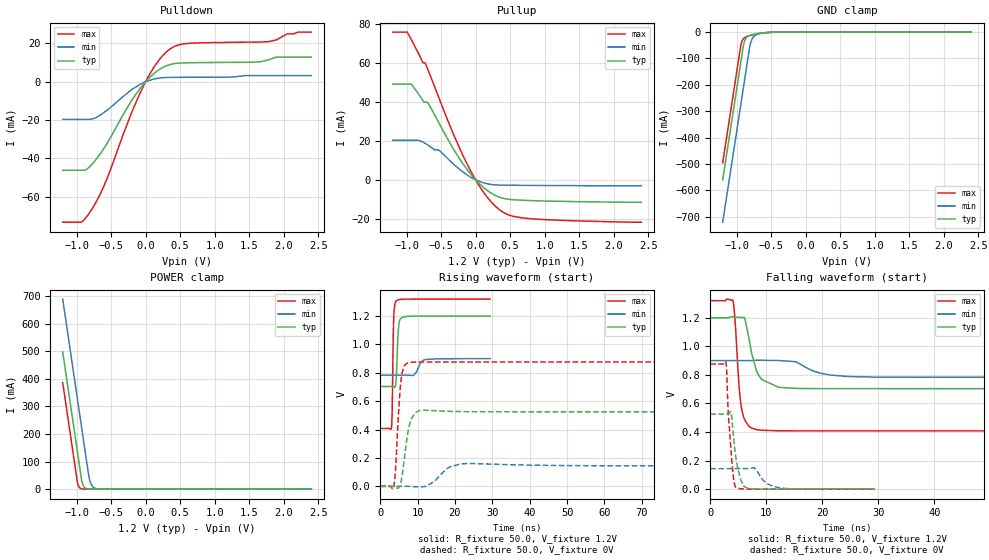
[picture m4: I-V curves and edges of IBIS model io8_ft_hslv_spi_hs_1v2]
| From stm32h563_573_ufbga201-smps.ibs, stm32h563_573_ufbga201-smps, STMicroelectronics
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[Model]   io8_ft_hslv_spi_hs_1v2
Model_type I/O
Polarity   Non-Inverting
Enable   Active-Low
| CAP_THRESHOLD on pad IOFT is "UDTCAPC" :
| Rising=20.0% of vddiom   Falling=80.0% of vddiom
| C_comp min and max val. don't necessarily correlate with the min and max pvt
| but are the smallest and greatest pad capacitance found.
| var   typ   min   max
C_comp   4.03050pF  3.93195pF  4.03600pF
|C_comp_pullup   2.46575pF  2.28000pF  2.18940pF
|C_comp_pulldown   1.56475pF  1.65195pF  1.84660pF
Vinl = 270.0mV
Vinh = 924.0mV
Vmeas = 600.0mV   | Reference voltage for timing measurements
Cref  = 50.0pF   | Timing specification test load capacitance value
Rref  = 100.0MOhm   | Timing specification test load resistance value
Vref  = 600.0mV   | Timing specification test load voltage
[Model Spec]
| TIME_THRESHOLD on pin ZIV11 is "CMOS" :
| Rising=40.0% of vdd   Falling=60.0% of vdd
Vinl 447.80000mV 344.80000mV 489.80000mV
Vinh 733.20000mV 535.20000mV 813.20000mV
| variable   typ   min   max
[Temperature Range] 25.0 125.0 -40.0
| variable   typ   min   max
[Voltage Range] 1.2V 900.0mV 1.32V
| variable   typ   min   max
[POWER Clamp Reference] 1.2V 900.0mV 1.32V
| variable   typ   min   max
[GND Clamp Reference] 0V 0V 0V
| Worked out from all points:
|   slope of the pulldown table from 0 to 0.18 V, typ, clamps not added: 30.6 ohm
|   slope of the pullup table from 0 to 0.18 V, typ, clamps not added: 31.3 ohm
|   GND clamp passes 1 mA (typ) near -0.52 V on its own axis
|   POWER clamp passes 1 mA (typ) near -0.84 V on its own axis
|   rising waveform, R_fixture 50.0, V_fixture 1.2V: 20-80 % time 487ps typ, 1.34ns min, 319ps max; typ from 0.704 V to 1.2 V
|   falling waveform, R_fixture 50.0, V_fixture 1.2V: 20-80 % time 1.88ns typ, 4.4ns min, 987ps max; typ from 1.2 V to 0.704 V
|   rising waveform, R_fixture 50.0, V_fixture 0V: 20-80 % time 1.69ns typ, 3.33ns min, 1.17ns max; typ from 0 V to 0.525 V
|   falling waveform, R_fixture 50.0, V_fixture 0V: 20-80 % time 1.14ns typ, 2.16ns min, 862ps max; typ from 0.525 V to 0 V
[POWER Clamp]
-1.2V     497.8mA    689.2mA    386.5mA
-990mV    140.8mA    332.2mA    29.53mA
-980mV    123.8mA    315.2mA    17.95mA
-960mV    89.81mA    281.2mA    6.634mA
-930mV    38.81mA    230.2mA    1.49mA
-900mV    12.07mA    179.2mA    334.8uA
-870mV    3.756mA    128.2mA    75.22uA
-820mV    536.4uA    44.98mA    6.246uA
-790mV    166.9uA    18.76mA    1.403uA
-750mV    35.18uA    5.846mA    191.9nA
-590mV    70.47nA    54.99uA    202.5pA
2.4V      0A         0A         0A
[GND Clamp]
-1.2V     -559.6mA   -720.6mA   -495.5mA
-940mV    -117.6mA   -278.6mA   -53.46mA
-930mV    -100.6mA   -261.6mA   -41.27mA
-900mV    -50.49mA   -210.6mA   -24.86mA
-880mV    -31.4mA    -176.6mA   -20.57mA
-850mV    -18.9mA    -125.6mA   -16.88mA
-810mV    -12.57mA   -58.3mA    -13.49mA
-780mV    -10.11mA   -29.57mA   -11.38mA
-740mV    -7.754mA   -14.31mA   -8.91mA
-640mV    -3.713mA   -4.821mA   -4.078mA
-390mV    -82.2uA    -288.6uA   -29.73uA
2.4V      3.859nA    727.3nA    172.3pA
| variable   typ   min   max
[Pullup Reference] 1.2V 900.0mV 1.32V
| variable   typ   min   max
[Pulldown Reference] 0V 0V 0V
[Pullup]
-1.2V     49.2mA     20.32mA    75.95mA
-990mV    49.2mA     20.32mA    75.95mA
-930mV    49.2mA     20.32mA    72.12mA
-750mV    40.06mA    19.16mA    60.18mA
-690mV    39.51mA    17.84mA    56.61mA
-530mV    29.17mA    15.19mA    42.06mA
-330mV    16.34mA    8.387mA    24.22mA
-80mV     3.3mA      1.496mA    5.118mA
140mV     -4.679mA   -1.778mA   -7.6mA
350mV     -8.973mA   -2.692mA   -15.46mA
760mV     -10.63mA   -2.872mA   -19.88mA
2.4V      -11.52mA   -3.045mA   -21.79mA
[Pulldown]
-1.2V     -46.17mA   -19.62mA   -73.27mA
-930mV    -46.17mA   -19.62mA   -73.17mA
-770mV    -42.8mA    -19.41mA   -66.04mA
-570mV    -32.88mA   -15.18mA   -51.58mA
-200mV    -9.658mA   -4.084mA   -15.89mA
-80mV     -3.488mA   -1.363mA   -5.887mA
140mV     4.817mA    1.546mA    8.585mA
340mV     8.782mA    2.251mA    16.66mA
540mV     9.805mA    2.305mA    19.74mA
1.79V     11.49mA    3.197mA    20.93mA
2.05V     12.83mA    3.197mA    24.95mA
2.4V      12.83mA    3.197mA    25.89mA
[Ramp]
dV/dt_r 315.18671mV/1.69216ns 86.16808mV/3.07186ns 525.78845mV/1.17248ns
dV/dt_f 297.79719mV/1.86448ns 69.92389mV/4.24582ns 547.13924mV/985.33046ps
R_load = 50.0
| Removed startup time: 0s 0s 0s  .
| Removed end time: 29.4ns.
[Rising Waveform]
R_fixture   = 50.0
V_fixture   = 1.2V
V_fixture_min = 900.0mV
V_fixture_max = 1.32V
0s        703.7mV    783.5mV    408.1mV
3ns       704mV      783.4mV    414mV
3.2ns     704.2mV    783.5mV    552.4mV
3.45ns    703.3mV    783.5mV    1.03V
3.6ns     701.2mV    783.5mV    1.184V
4.25ns    758.2mV    783.5mV    1.307V
4.95ns    1.136V     783.5mV    1.316V
6ns       1.192V     783.6mV    1.319V
12ns      1.2V       892.9mV    1.32V
29.4ns    1.2V       900mV      1.32V
| Removed startup time: 0s 0s 0s  .
| Removed end time: 149.4ns.
[Falling Waveform]
R_fixture   = 50.0
V_fixture   = 1.2V
V_fixture_min = 900.0mV
V_fixture_max = 1.32V
0s        1.2V       900mV      1.32V
4.05ns    1.207V     900mV      1.32V
4.4ns     1.205V     900mV      1.193V
5.15ns    1.202V     900mV      716.4mV
5.65ns    1.202V     900mV      550.6mV
6.2ns     1.188V     900mV      481.1mV
8.55ns    803.3mV    902.7mV    414.9mV
12.2ns    712.9mV    900.7mV    408.8mV
27.45ns   703.7mV    785.7mV    408.1mV
149.4ns   703.7mV    783.5mV    408.1mV
| Removed startup time: 0s 0s 0s  .
| Removed end time: 149.4ns.
[Rising Waveform]
R_fixture   = 50.0
V_fixture   = 0V
V_fixture_min = 0V
V_fixture_max = 0V
0s        166.4nV    850.8nV    114.3nV
3.6ns     322.3uV    -4.011uV   -4.146mV
4ns       -4.023mV   -2.261uV   88.4mV
5ns       -6.828mV   488.5nV    563.8mV
5.6ns     38.14mV    -4.334uV   755.2mV
6.4ns     186.3mV    -9.598uV   845.8mV
7.7ns     420.1mV    121.7uV    872.6mV
10.4ns    533.7mV    -5.243mV   876.1mV
23.7ns    526.4mV    160.9mV    876.2mV
149.4ns   525.3mV    143.6mV    876.3mV
| Removed startup time: 0s 0s 0s  .
| Removed end time: 29.4ns.
[Falling Waveform]
R_fixture   = 50.0
V_fixture   = 0V
V_fixture_min = 0V
V_fixture_max = 0V
0s        525.3mV    143.6mV    876.3mV
2.8ns     525.3mV    143.6mV    890.3mV
3.25ns    526.7mV    143.6mV    506.1mV
3.75ns    529.9mV    143.6mV    244.9mV
4.2ns     345.9mV    143.6mV    62.85mV
4.65ns    199.8mV    143.6mV    10.18mV
5.4ns     69.34mV    143.6mV    2.84mV
6.6ns     6.961mV    143.8mV    1.009mV
12.6ns    202uV      8.242mV    118.6uV
29.4ns    2.57uV     11.5uV     393.6nV
